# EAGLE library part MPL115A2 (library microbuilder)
MPL115A2 I2C Barometric Pressure Sensor (50-115 kPa/7.25-16.68 PSI) - LGA8 Package Digikey: MPL115A2T1CT-ND
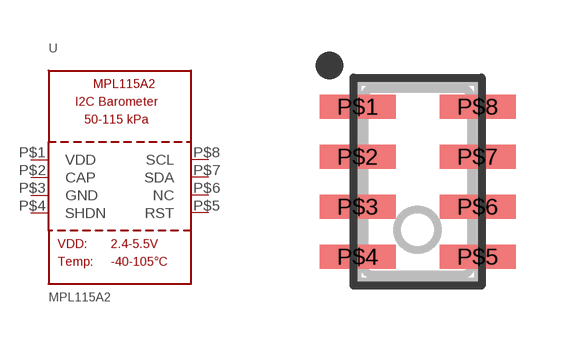
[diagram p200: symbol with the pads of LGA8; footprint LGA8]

Designator prefix U

## MPL115A2  [LGA8]
P$1  VDD  pwr
P$2  CAP
P$3  GND  pwr
P$4  SHDN
P$5  RST
P$6  NC  nc
P$7  SDA
P$8  SCL

## Footprint LGA8 (pad centres in mm)
LGA8 3x5mm 1.25mm Pitch Source: http://www.freescale.com/files/sensors/doc/data_sheet/MPL115A2.pdf
smd 1.9 x 0.6: P$1 -1.5,1.875; P$2 -1.5,0.625; P$3 -1.5,-0.625; P$4 -1.5,-1.875; P$5 1.5,-1.875; P$6 1.5,-0.625; P$7 1.5,0.625; P$8 1.5,1.875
